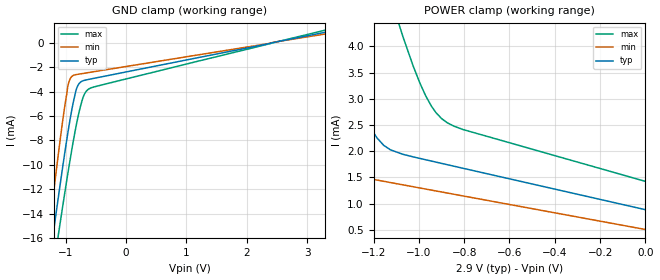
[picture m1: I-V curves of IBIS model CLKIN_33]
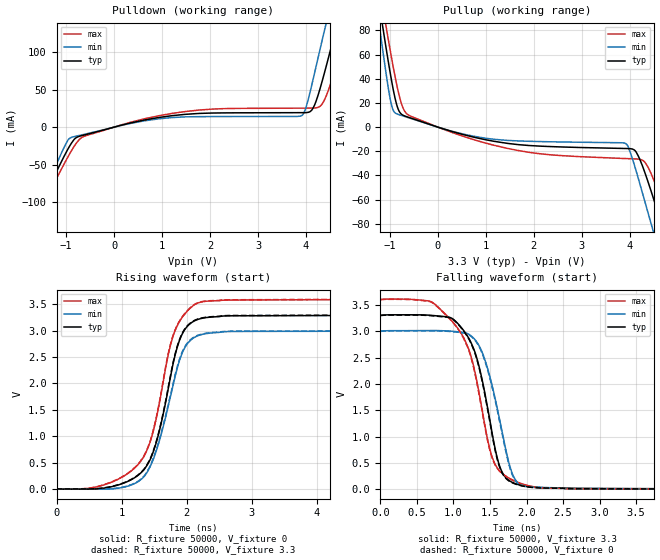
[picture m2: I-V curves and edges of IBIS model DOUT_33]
| TEXAS INSTRUMENTS INCORPORATED
| High Performance Analog Group
| IBIS Model of ADS5424
| 14-Bit, 105MSPS ADC
| This file contains package information for the following:
|  HTQFP 52-pin (PAP) package as [Component] ADS5424_PAP
| This device can be powered at the following Vccs:
|  3.3 volt Vcc
| This file provides unique models under the [Model Selector] for each Vcc.
| For operation at a specific Vcc, select the appropriate model after each
| [Model Selector] keyword.
[IBIS Ver]   3.2
[Comment char]  |_char
[File Name]   ads5424.ibs
[File Rev]   4.0 |
[Date]   December 21, 2004
[Source]   Data created from TI-SPICE simulations at TI-HPA.
[Notes]   The following is an IBIS list for the ADS5424.
##notes##|
[Disclaimer] Property of Texas Instruments Incorporated.  Unauthorized
   reproduction and/or distribution is strictly prohibited.
   This product is protected under copyright law.
   Created  2004, (C) Copyright  2004, Texas Instruments
   Incorporated, All Rights Reserved
   UNLESS THERE IS A SIGNED, WRITTEN AGREEMENT TO THE
   CONTRARY, TEXAS INSTRUMENTS (TI) IS PROVIDING THE IBIS
   MODELS  AND WITHOUT ANY WARRANTY, EXPRESSED OR
   IMPLIED.  TI assumes no liability for:
   1) the accuracy of the IBIS models provided to your
   company;
   2) the proper functioning of these IBIS Models in your
   design or for any resulting applications; or
   3) infringement of patents, copyrights or intellectual
   property rights resulting from your use of these IBIS
   models.
   TI provides IBIS Models as a service to our customers.
   You and your company shall not distribute, sell or give
   these models to anyone else without prior written
   permission from TI.
   TI reserves the right to make changes to our products or
   to discontinue any semiconductor product or service
   without notice, and advises our customers to obtain the
   latest version of relevant information to verify, before
   placing orders, that the information being relied on is
   current.
   Please be aware that your receipt and use of the IBIS
   information provided shall serve as acceptance of these
   terms and conditions.  If you do not accept these terms,
   you should return or destroy the IBIS models and any
   other accompanying information immediately.
| Component ADS5424_PAP 52-pin HTQFP
[Component]   ADS5424_PAP
[Manufacturer]   Texas Instruments, Inc.
[Package]
|   typ   min   max
R_pkg   9.337e-02   5.032e-02   1.437e-01
L_pkg   2.475e-09   1.898e-09   2.990e-09
C_pkg   5.413e-13   4.269e-13   6.693e-13
[Pin]   signal_name   model_name   R_pin   L_pin   C_pin
1   DRVDD   POWER   7.188e-02   2.564e-09   6.021e-13
2   GND   NC   6.888e-02   2.435e-09   6.620e-13
3   VERF   NC   1.212e-01   2.589e-09   4.555e-13
4   GND   NC   1.143e-01   2.459e-09   4.453e-13
5   CLK   CLKIN   1.070e-01   2.328e-09   4.383e-13
6   CLK_b   CLKIN   9.791e-02   2.180e-09   4.413e-13
7   GND   NC   5.108e-02   1.910e-09   5.711e-13
8   AVDD   NC   5.032e-02   1.919e-09   5.497e-13
9   AVDD   POWER   5.049e-02   1.946e-09   5.392e-13
10   GND   GND   5.214e-02   2.014e-09   5.515e-13
11   AIN   NC   1.045e-01   2.364e-09   4.449e-13
12   AIN_b   NC   1.229e-01   2.648e-09   4.658e-13
13   GND   NC   7.226e-02   2.579e-09   6.445e-13
14   AVDD   NC   7.692e-02   2.683e-09   6.248e-13
15   GND   NC   7.382e-02   2.552e-09   6.519e-13
16   AVDD   NC   7.128e-02   2.477e-09   6.347e-13
17   GND   NC   7.149e-02   2.446e-09   6.294e-13
18   AVDD   NC   7.176e-02   2.421e-09   6.282e-13
19   GND   NC   7.243e-02   2.413e-09   6.457e-13
20   C1   NC   7.374e-02   2.417e-09   6.660e-13
21   GND   NC   7.361e-02   2.439e-09   6.492e-13
22   AVDD   NC   7.392e-02   2.469e-09   6.382e-13
23   GND   NC   7.450e-02   2.513e-09   6.460e-13
24   C2   NC   7.588e-02   2.580e-09   6.591e-13
25   GND   NC   7.768e-02   2.638e-09   6.693e-13
26   AVDD   NC   7.854e-02   2.720e-09   6.314e-13
27   GND   GND   7.136e-02   2.558e-09   6.389e-13
28   AVDD   NC   6.525e-02   2.360e-09   6.411e-13
29   GND   NC   5.890e-02   2.200e-09   5.980e-13
30   AVDD   NC   5.548e-02   2.088e-09   5.702e-13
31   DNC   NC   9.832e-02   2.212e-09   4.307e-13
32   OVR   DOUT   9.479e-02   2.140e-09   4.374e-13
33   DRVDD   POWER   5.050e-02   1.898e-09   5.563e-13
34   GND   GND   5.060e-02   1.925e-09   5.528e-13
35   DMID   NC   9.938e-02   2.223e-09   4.335e-13
36   D0   DOUT   1.087e-01   2.381e-09   4.415e-13
37   D1   DOUT   1.167e-01   2.528e-09   4.507e-13
38   D2   DOUT   1.253e-01   2.674e-09   4.616e-13
39   D3   DOUT   1.349e-01   2.870e-09   4.269e-13
40   D4   DOUT   1.419e-01   2.966e-09   4.302e-13
41   D5   DOUT   1.391e-01   2.864e-09   4.696e-13
42   GND   GND   7.214e-02   2.488e-09   6.367e-13
43   DRVDD   POWER   7.157e-02   2.439e-09   6.076e-13
44   D6   DOUT   1.366e-01   2.736e-09   4.608e-13
45   D7   DOUT   1.372e-01   2.720e-09   4.683e-13
46   D8   DOUT   1.374e-01   2.699e-09   4.926e-13
47   D9   DOUT   1.376e-01   2.726e-09   4.688e-13
48   D10   DOUT   1.378e-01   2.752e-09   4.590e-13
49   D11   DOUT   1.384e-01   2.792e-09   4.616e-13
50   D12   DOUT   1.395e-01   2.844e-09   4.656e-13
51   D13   DOUT   1.418e-01   2.903e-09   4.706e-13
52   DRY   DOUT   1.437e-01   2.990e-09   4.312e-13
| NOTE:  The [Diff Pin] section is commented out because the ibischk3 program
|   currently flags it as an Error when it shouldn't
| [Diff Pin]  inv_pin   vdiff   tdelay_typ
|5   6   50m   NA
| Model CLKIN
[Model Selector]   CLKIN
CLKIN_33   3.3 volt Vcc
| Model DOUT
[Model Selector]   DOUT
DOUT_33   3.3 volt Vcc
| Models and submodels in the file (2): CLKIN_33 (Input), DOUT_33 (Output)
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[Model]   CLKIN_33
Model_type  Input
| variable   typ   min   max
C_comp   0.79pF   0.21pF   1.71pF
[Temperature Range]   40   -40   100
| Ambient temperature   25   -40   85
[Voltage range]   2.9   2.9   2.9
[GND Clamp]
| CLKIN_33
|   Voltage   I(typ)   I(min)   I(max)
-2.9V     -68.32mA   -68.96mA   -68.94mA
-1.325V   -20.01mA   -17.45mA   -22.59mA
-1.215V   -16.04mA   -12.94mA   -18.9mA
-1.165V   -14.25mA   -10.9mA    -17.24mA
-1.11V    -12.3mA    -8.715mA   -15.42mA
-965mV    -7.444mA   -3.604mA   -10.78mA
-930mV    -6.39mA    -2.994mA   -9.713mA
-880mV    -5.043mA   -2.68mA    -8.259mA
-810mV    -3.634mA   -2.579mA   -6.417mA
-725mV    -3.127mA   -2.509mA   -4.678mA
-600mV    -2.967mA   -2.409mA   -3.728mA
3.3V      884.4uA    745uA      1.061mA
[POWER Clamp]
| CLKIN_33
|   Voltage   I(typ)   I(min)   I(max)
-2.9V     34.26mA    9.537mA    60.57mA
-1.675V   8.038mA    4.323mA    10.17mA
-1.475V   5.525mA    2.137mA    9.528mA
-1.425V   4.875mA    1.779mA    9.049mA
-1.385V   4.361mA    1.639mA    8.578mA
-1.225V   2.549mA    1.482mA    6.362mA
-1.185V   2.255mA    1.45mA     5.783mA
-1.125V   2.026mA    1.402mA    4.928mA
-1.07V    1.941mA    1.358mA    4.182mA
-970mV    1.838mA    1.279mA    3.058mA
-875mV    1.744mA    1.203mA    2.544mA
-39.59fV  884.4uA    506.6uA    1.425mA
[Model]   DOUT_33
Model_type  Output
Vref =   0
Rref =   50000
Cref =   3p
Vmeas =   1.5
| variable   typ   min   max
C_comp   0.96pF   0.56pF   1.59pF
| C_pullup   0.97pF   0.56pF   1.31pF
| C_pulldown   0.96pF   0.57pF   1.59pF
[Temperature Range]   40   -40   100
| Ambient temperature   25   -40   85
[Voltage range]   3.3   3   3.6
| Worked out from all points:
|   slope of the pulldown table from 0 to 0.495 V, typ, clamps not added: 64.7 ohm
|   slope of the pullup table from 0 to 0.495 V, typ, clamps not added: 85.4 ohm
|   rising waveform, R_fixture 50000, V_fixture 0: 20-80 % time 370ps typ, 381ps min, 402ps max; typ from 0 V to 3.29 V
|   falling waveform, R_fixture 50000, V_fixture 3.3: 20-80 % time 303ps typ, 297ps min, 367ps max; typ from 3.3 V to 0.004 V
|   rising waveform, R_fixture 50000, V_fixture 3.3: 20-80 % time 370ps typ, 381ps min, 402ps max; typ from 0.004 V to 3.3 V
|   falling waveform, R_fixture 50000, V_fixture 0: 20-80 % time 303ps typ, 297ps min, 367ps max; typ from 3.29 V to 0 V
[Pulldown]
| DOUT_33
|   Voltage   I(typ)   I(min)   I(max)
-3.3V     -284.4mA   -285.6mA   -287.4mA
-1.805V   -136.8mA   -135mA     -141.9mA
-1.045V   -39.26mA   -27.32mA   -49.53mA
-860mV    -18.71mA   -13.07mA   -28.42mA
-630mV    -10.59mA   -9.706mA   -12.34mA
1.205V    15.27mA    12.77mA    18.28mA
3.91V     19.3mA     15.3mA     25.34mA
4.15V     25.66mA    64.35mA    25.43mA
4.425V    82.21mA    139.8mA    42.2mA
4.66V     139.7mA    199.4mA    88.93mA
4.87V     189.6mA    247.3mA    136.4mA
6.6V      433.1mA    454.2mA    411.1mA
[Pullup]
| DOUT_33
|   Voltage   I(typ)   I(min)   I(max)
-1.8V     240.6mA    236.1mA    249.2mA
-1.285V   117.7mA    102.8mA    132.1mA
-1.145V   82.07mA    62.76mA    98.8mA
-975mV    40.8mA     19.86mA    59.55mA
-860mV    18.89mA    11.05mA    35.69mA
-635mV    8.446mA    8.093mA    10.61mA
580mV     -6.678mA   -6.162mA   -8.254mA
3.895V    -17.65mA   -13.25mA   -25.97mA
4.135V    -20.72mA   -36.54mA   -26.33mA
4.48V     -57.3mA    -84.73mA   -41.76mA
4.865V    -105.1mA   -135.4mA   -84.56mA
6.6V      -278.5mA   -299.5mA   -263.4mA
[Ramp]
| DOUT_33
| variable   typ   min   max
dV/dt_r   1.98/3.77E-10   1.80/3.87E-10   2.16/4.09E-10
dV/dt_f   1.98/3.08E-10   1.80/3.00E-10   2.16/3.73E-10
R_load = 50000
[Rising Waveform]
| DOUT_33
R_fixture =   50000
C_fixture =   0
L_fixture =   0
V_fixture =   0
V_fixture_min = 0
V_fixture_max = 0
|   Time   V(typ)   V(min)   V(max)
0s        1.562nV    1.335nV    282.5nV
800ps     29.6mV     -3.062mV   105.9mV
1.34ns    359.4mV    227.3mV    610.2mV
1.445ns   575.1mV    440.7mV    918.7mV
1.55ns    960.1mV    791.3mV    1.442V
1.72ns    1.928V     1.594V     2.57V
1.82ns    2.531V     2.125V     2.999V
2.005ns   3.078V     2.746V     3.367V
2.305ns   3.25V      2.946V     3.559V
29.99ns   3.295V     2.995V     3.595V
[Falling Waveform]
| DOUT_33
R_fixture =   50000
C_fixture =   0
L_fixture =   0
V_fixture =   3.3
V_fixture_min = 3
V_fixture_max = 3.6
|   Time   V(typ)   V(min)   V(max)
0s        3.3V       3V         3.6V
725ps     3.297V     3.012V     3.535V
1.005ns   3.219V     2.995V     3.153V
1.265ns   2.706V     2.884V     2.398V
1.37ns    2.22V      2.673V     1.686V
1.5ns     1.3V       2.13V      749.8mV
1.665ns   327.4mV    1.1V       303.6mV
1.85ns    103.2mV    174mV      147.7mV
2.19ns    28.2mV     35.06mV    28.76mV
29.99ns   3.72mV     3.715mV    3.529mV
[Rising Waveform]
| DOUT_33
R_fixture =   50000
C_fixture =   0
L_fixture =   0
V_fixture =   3.3
V_fixture_min = 3
V_fixture_max = 3.6
|   Time   V(typ)   V(min)   V(max)
0s        3.718mV    3.712mV    3.527mV
800ps     33.96mV    1.406mV    110.1mV
1.34ns    368.1mV    237.6mV    619.1mV
1.445ns   588.4mV    456.4mV    932.6mV
1.55ns    979.2mV    812.6mV    1.462V
1.715ns   1.92V      1.595V     2.559V
1.815ns   2.526V     2.127V     2.996V
2ns       3.081V     2.752V     3.368V
2.3ns     3.256V     2.952V     3.564V
29.99ns   3.3V       3V         3.6V
[Falling Waveform]
| DOUT_33
R_fixture =   50000
C_fixture =   0
L_fixture =   0
V_fixture =   0
V_fixture_min = 0
V_fixture_max = 0
|   Time   V(typ)   V(min)   V(max)
0s        3.295V     2.995V     3.595V
725ps     3.291V     3.005V     3.529V
1.09ns    3.09V      2.975V     2.984V
1.265ns   2.691V     2.872V     2.377V
1.37ns    2.195V     2.655V     1.658V
1.5ns     1.268V     2.101V     730.3mV
1.66ns    325mV      1.096V     303.1mV
1.85ns    96.73mV    158.9mV    142.9mV
2.185ns   24.16mV    30.61mV    25.47mV
29.99ns   2.175uV    2.822uV    1.936uV
